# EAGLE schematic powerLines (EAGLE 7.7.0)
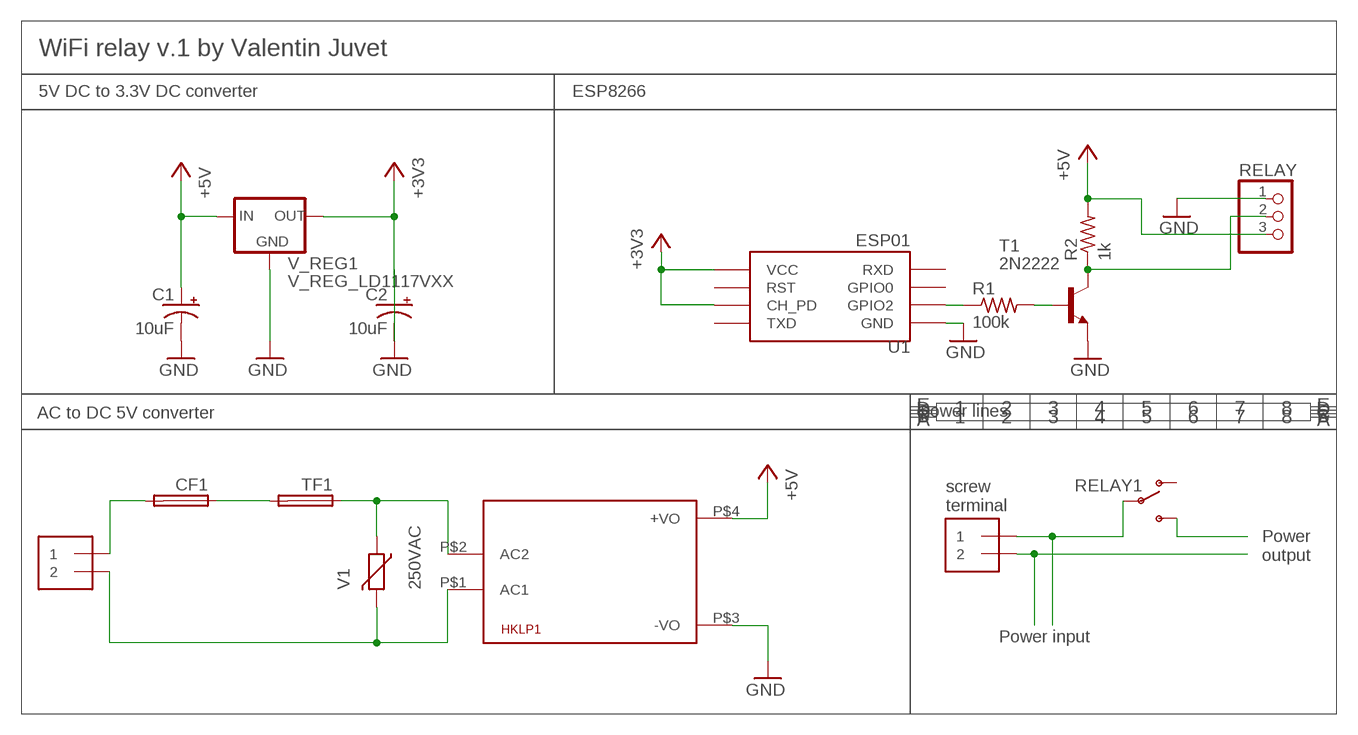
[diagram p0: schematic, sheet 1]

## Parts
C1  10uF  10UF-POLAR-RADIAL-2.5MM-25V-20%  [CPOL-RADIAL-2.5MM-5MM]
C2  10uF  10UF-POLAR-RADIAL-2.5MM-25V-20%  [CPOL-RADIAL-2.5MM-5MM]
CF1  TE5  [TE5]
HKLP1  HKLPM01  [HKLPM01]
J1  1X2-3.5MM  [1X2-3.5MM]
J2  1X2-3.5MM  [1X2-3.5MM]
R1  100k  R-US_0207/10  [0207/10]
R2  1k  R-US_0207/10  [0207/10]
RELAY  PINHD-1X3CB  [1X03-CLEANBIG]
RELAY1  SWITCH-SPDTPTH2  [SWITCH-DPDT]
T1  2N2222  [TO92-EBC-OVAL]
TF1  TE5  [TE5]
U1  ESP01  [ESP01]
V1  250VAC  VARISTOR-7,5  [R-7,5]
V_REG1  V_REG_LD1117VXX  [78XXL]

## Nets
+3V3: C2.1(+) U1.CH_PD U1.VCC V_REG1.GND(OUT)
+5V: C1.1(+) HKLP1.P$4(+VO) R2.2 RELAY.3 V_REG1.OUT(IN)
GND: C1.2(-) C2.2(-) HKLP1.P$3(-VO) RELAY.1 T1.E U1.GND V_REG1.IN(GND)
N$1 [250AC]: CF1.2 J1.1
N$2 [250AC]: CF1.1 TF1.2
N$3 [250AC]: HKLP1.P$1(AC1) J1.2 V1.2
N$4 [250AC]: HKLP1.P$2(AC2) TF1.1 V1.1
N$5: R1.1 U1.GPIO2
N$6: R1.2 T1.B
N$7: R2.1 RELAY.2 T1.C
N$8: J2.2
N$9: J2.1 RELAY1.2(P)
N$10: RELAY1.3(S)
Unconnected: RELAY1.1(O) U1.GPIO0 U1.RST U1.RX(RXD) U1.TX(TXD)

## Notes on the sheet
- WiFi relay v.1 by Valentin Juvet
- 5V DC to 3.3V DC converter | ESP8266
- AC to DC 5V converter | power lines
- screw
  terminal
- Power
  output
- Power input

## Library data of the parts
C1 C2 = SparkFun-Capacitors:10UF-POLAR: 10.0µF polarized capacitors; PROD_ID: CAP-08440
CF1 TF1 = fuse:TE5: FUSE; OC_FARNELL: unknown; OC_NEWARK: unknown
HKLP1 = HKLPM01:HKLPM01
J1 J2 = adafruit:1X2: 3.5mm Terminal block
R1 R2 = adafruit:R-US_: RESISTOR, American symbol
RELAY = adafruit:PINHD-1X3: PIN HEADER
RELAY1 = SparkFun-Retired:SWITCH-SPDT: SPDT Switch Simple slide switch, Spark Fun Electronics SKU : COM-00102 DPDT SMT slide switch, AYZ0202, SWCH-08179
T1 = adafruit:2N2222: NPN TRANSISTOR Big oval pads
U1 = ESP8266:ESP01: ESP8266 Wifi module 01
V1 = varistor:VARISTOR: VARISTOR
V_REG1 = SparkFun-IC-Power:V_REG_LD1117VXX: LD1117VXX voltage regulator. We carry the 3.3V version (COM-00526) in TO-220 package.

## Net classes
0 default: width 0.305 mm, drill 0.508 mm, clearance 0.254 mm
1 250AC: width 1.27 mm, drill 2.032 mm, clearance 1.016 mm

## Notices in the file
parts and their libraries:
SparkFun-IC-Power: Licensing: Creative Commons ShareAlike 4.0 International - https://creativecommons.org/licenses/by-sa/4.0
